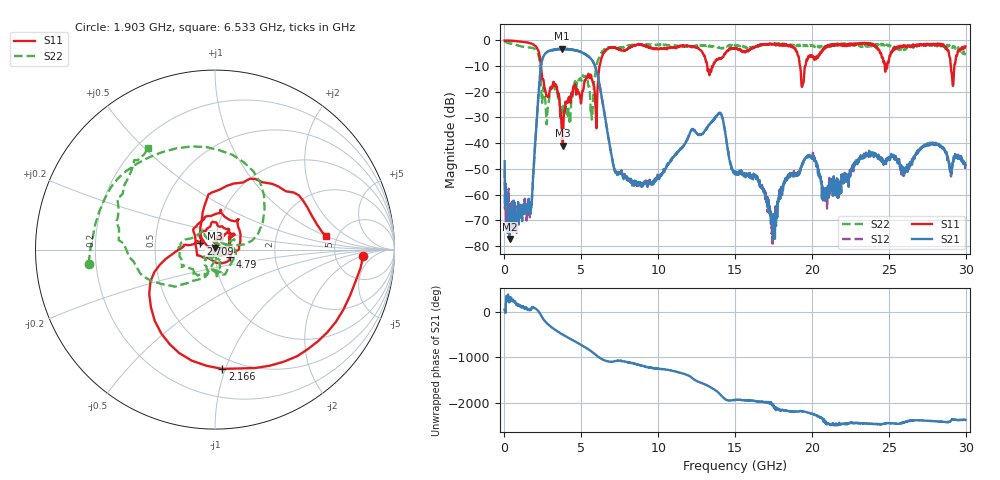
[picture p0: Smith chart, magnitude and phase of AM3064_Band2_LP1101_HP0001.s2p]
# Hz S DB R 50.0
!freq dBS11 angS11 dBS21 angS21 dBS12 angS12 dBS22 angS22
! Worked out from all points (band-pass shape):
!   1600 points, 10 MHz to 29.98 GHz, reference 50 ohm
!   highest |S21| = -3.25 dB at 3.759 GHz (marker M1); lowest = -77.3 dB at 347.4 MHz (marker M2)
!   |S21| within 3 dB of the highest: 2.536 GHz to 5.471 GHz (2.935 GHz wide, 73.3 % of centre)
!   lowest |S11| = -41.0 dB at 3.796 GHz (marker M3), VSWR 1.02, Z = 50.1 + j0.882 ohm
!   |S11| at or under -10 dB: 2.373 GHz to 6.19 GHz (3.818 GHz wide, 89.2 % of centre); 13.19 GHz to 13.56 GHz (375.6 MHz wide, 2.81 % of centre); 19.23 GHz to 19.58 GHz (353.9 MHz wide, 1.82 % of centre)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
!   |S22| runs from -32.7 to -0.2 dB; largest |S21 - S12| = 0.021
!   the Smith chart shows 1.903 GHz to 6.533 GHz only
!   S11 on the Smith chart (normalised r, x): 1.903 GHz: 10, -2; 2.166 GHz: 0.41, -0.98; 2.709 GHz: 0.85, +0.06; 4.79 GHz: 1.18, -0.10; 6.533 GHz: 4.06, +1.03
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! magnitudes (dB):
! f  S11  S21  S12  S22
! 10 MHz  -0.1  -47.0  -50.2  -0.2
! 347.4 MHz  -0.1  -77.3  -71.9  -1.2
! 1.584 GHz  -1.0  -61.7  -63.9  -2.7
! 1.903 GHz  -1.6  -49.1  -49.6  -3.0
! 2.166 GHz  -3.5  -25.2  -25.1  -4.8
! 2.709 GHz  -21.0  -4.9  -4.8  -29.4
! 3.759 GHz  -34.4  -3.2  -3.3  -27.9
! 3.796 GHz  -41.0  -3.3  -3.3  -28.2
! 4.79 GHz  -20.6  -4.1  -4.1  -16.3
! 5.015 GHz  -22.1  -4.6  -4.7  -15.7
! 5.689 GHz  -15.1  -7.6  -7.7  -30.8
! 5.971 GHz  -33.8  -11.5  -11.5  -10.3
! 6.533 GHz  -4.1  -29.6  -29.4  -3.4
! 7.283 GHz  -3.1  -51.2  -51.7  -2.7
! 10 GHz  -3.4  -53.3  -52.6  -1.8
! 13.97 GHz  -6.8  -28.6  -28.2  -2.8
! 15 GHz  -2.9  -52.1  -51.8  -1.9
! 17.44 GHz  -1.4  -68.5  -80.1  -1.5
! 19.99 GHz  -5.9  -45.2  -45.5  -1.8
! 20.85 GHz  -3.0  -61.6  -62.9  -2.5
! 25 GHz  -8.0  -45.4  -46.0  -1.7
! 29.98 GHz  -2.3  -48.4  -48.3  -4.6
